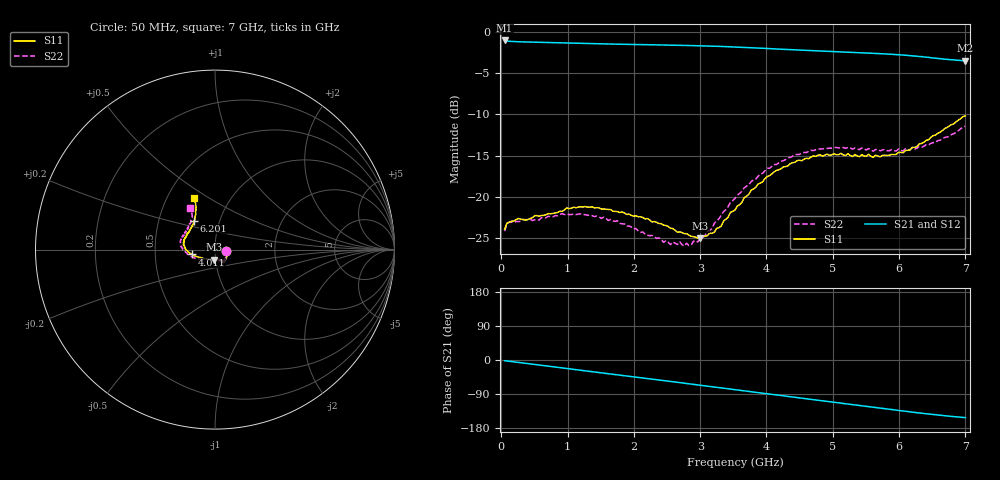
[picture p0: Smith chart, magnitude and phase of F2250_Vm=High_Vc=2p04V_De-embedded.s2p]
! Integrated Device Technology
! Corporate Headquarters
! 6024 Silver Creek Valley Road
! San Jose, CA 95138  USA
! Phone:  1-408-284-8200
! Toll Free:  1-800-223-1366
! Webpage:  http://www.idt.com/
! Timing and RF Division
! 515 Groton Road, Suite 102
! Westford, MA 01886-6024
! Device:  F2250
! Description: Voltage Variable RF Attenuator
! Frequency:  50.0 -  6000.00 MHz
! Package:  3x3 mm Thin QFN Plastic Package: 16 pin
! Ports:  2 RF, 3 DC
!  Pin  1  = GND
!  Pin  2  = NC
!  Pin  3  = RF1  = Port 1
!  Pin  4  = NC
!  Pin  5  = GND
!  Pin  6  = GND
!  Pin  7  = GND
!  Pin  8  = GND
!  Pin  9  = NC
!  Pin 10  = RF2  = Port 2
!  Pin 11  = NC
!  Pin 12  = GND
!  Pin 13  = GND
!  Pin 14  = VCNTRL
!  Pin 15  = VDD
!  Pin 16  = VMODE
! Vcntrl:  2.040 Volts
! Vmode:  +3.300 Volts
! Vdd:  +3.30  Volts
! Current:  1.321 mA
! Data:  The device was measured on a the F2250 evaluation board which has
!  individual transmission lines to the RF pins.  Data was collected
!  using a calibrated network analyzer.  The evaluation board was
!  de-embedded using a TRL calibration technique.
!  The reference plane is the edge of the package pin.
! Misc:  SN 10
!  Action Tracker AT0258
! Date Measured:  2014-11-26
! Date:  2015-10-15  MJV
! Note:
!  Integrated Device Technology supplies this data as a sample of measured
!  data at the package pin for this product.  Your particular data for this
!  product may vary.
!  Data was taken at 25 degrees C.
!  Integrated Device Technology reserves the right to change this data at anytime.
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# GHz S dB R 50
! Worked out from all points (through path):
!   201 points, 50 MHz to 7 GHz, reference 50 ohm
!   highest |S21| = -1.00 dB at 50 MHz (marker M1); lowest = -3.5 dB at 7 GHz (marker M2)
!   group delay of S21, straight-line fit = 61.1 ps
!   lowest |S11| = -25.1 dB at 3.004 GHz (marker M3), VSWR 1.12, Z = 49.2 - j5.48 ohm
!   |S11| at or under -10 dB: start of sweep to end of sweep
!   |S22| runs from -26.0 to -11.4 dB; largest |S21 - S12| = 0.0019
!   S11 on the Smith chart (normalised r, x): 50 MHz: 1.13, -0.02; 4.011 GHz: 0.77, -0.04; 6.201 GHz: 0.75, +0.25; 7 GHz: 0.68, +0.43
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0.05  -24.00 -8.9  -1.00 -1.8  -1.00 -1.8  -24.20 -9.6
0.08475  -23.23 -8.1  -1.07 -2.5  -1.07 -2.5  -23.32 -8.5
0.1195  -23.11 -8.8  -1.10 -3.3  -1.10 -3.2  -23.13 -8.1
0.91875  -21.80 -44.9  -1.29 -21.0  -1.29 -21.1  -22.07 -48.0
1.2315  -21.27 -52.7  -1.36 -27.9  -1.36 -27.9  -22.18 -58.4
1.75275  -21.83 -59.6  -1.45 -39.1  -1.45 -39.1  -22.94 -66.1
2.37825  -23.28 -60.1  -1.54 -52.7  -1.54 -52.8  -25.03 -69.3
2.552  -23.86 -64.4  -1.56 -56.6  -1.57 -56.6  -25.85 -76.0
2.691  -24.29 -71.2  -1.59 -59.7  -1.59 -59.7  -25.49 -82.9
2.7605  -24.51 -73.1  -1.60 -61.3  -1.60 -61.3  -26.03 -87.1
3.00375  -25.08 -95.0  -1.65 -66.7  -1.65 -66.7  -24.98 -109.1
3.21225  -24.34 -117.0  -1.70 -71.4  -1.70 -71.4  -23.26 -127.5
3.525  -21.64 -144.7  -1.79 -78.5  -1.79 -78.5  -20.23 -146.2
3.76825  -19.21 -158.8  -1.88 -84.0  -1.88 -84.0  -18.18 -157.6
4.0115  -17.56 -168.3  -1.98 -89.4  -1.98 -89.4  -16.56 -167.3
4.4285  -15.82 179.8  -2.14 -98.6  -2.15 -98.6  -14.89 -180.0
4.7065  -15.05 172.5  -2.24 -104.8  -2.24 -104.8  -14.40 174.1
5.054  -14.91 164.2  -2.37 -112.4  -2.37 -112.5  -14.01 166.9
5.85325  -14.96 137.9  -2.67 -129.9  -2.67 -130.0  -14.42 147.9
6.20075  -14.01 125.8  -2.88 -137.6  -2.88 -137.7  -14.03 138.7
6.54825  -12.52 117.4  -3.15 -144.7  -3.15 -144.8  -13.40 127.3
7  -10.17 112.2  -3.47 -152.0  -3.48 -152.1  -11.42 121.0
